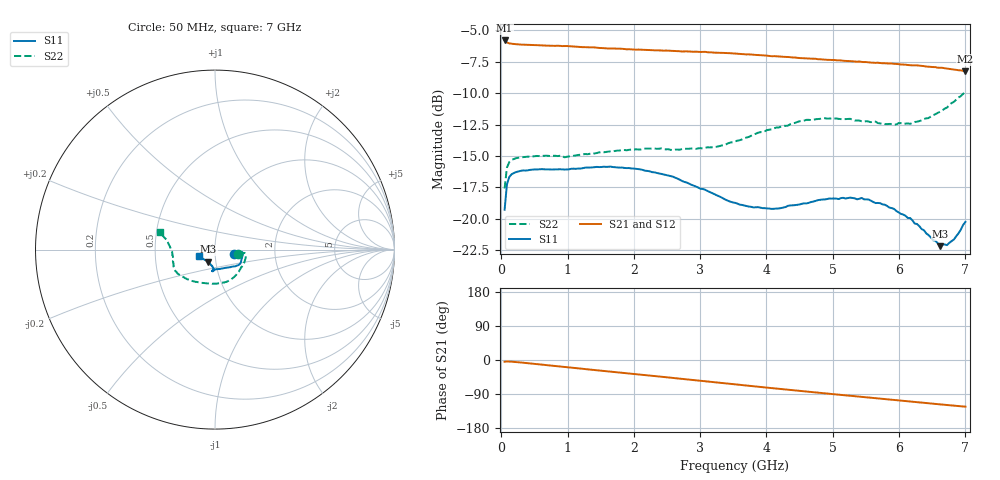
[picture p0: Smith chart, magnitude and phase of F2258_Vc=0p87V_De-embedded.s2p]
! Integrated Device Technology
! Corporate Headquarters
! 6024 Silver Creek Valley Road
! San Jose, CA 95138  USA
! Phone:  1-408-284-8200
! Toll Free:  1-800-223-1366
! Webpage:  http://www.idt.com/
! Timing and RF Division
! 515 Groton Road, Suite 102
! Westford, MA 01886-6024
! Device:  F2258
! Description: Voltage Variable RF Attenuator
! Frequency:  50.0 -  6000.00 MHz
! Package:  3x3 mm Thin QFN Plastic Package: 16 pin
! Ports:  2 RF, 2 DC
!  Pin  1  = NC
!  Pin  2  = NC
!  Pin  3  = RF2  = Port 2
!  Pin  4  = GND
!  Pin  5  = Vdd
!  Pin  6  = NC
!  Pin  7  = VCTRL
!  Pin  8  = NC
!  Pin  9  = GND
!  Pin 10  = RF1  = Port 1
!  Pin 11  = NC
!  Pin 12  = NC
!  Pin 13  = NC
!  Pin 14  = NC
!  Pin 15  = NC
!  Pin 16  = NC
! Vcntrl:  0.870 Volts
! Vdd:  +3.300 Volts
! Current:  1.145 mA
! Data:  The device was measured on a the F2258 evaluation board which has
!  individual transmission lines to the RF pins.  Data was collected
!  using a calibrated network analyzer.  The evaluation board was
!  de-embedded using a TRL calibration technique.
!  The reference plane is the edge of the package pin.
! Misc:  SN 10
!  Action Tracker AT0285
! Date Measured:  2014-12-10
! Date:  2016-01-13  MJV
! Note:
!  Integrated Device Technology supplies this data as a sample of measured
!  data at the package pin for this product.  Your particular data for this
!  product may vary.
!  Data was taken at 25 degrees C.
!  Integrated Device Technology reserves the right to change this data at anytime.
!Freq_(GHz)  S11M_(dB)  S11P_(deg)  S21M_(dB)  S21P_(deg)  S12M_(dB)  S12P_(deg)  S22M_(dB)  S22P_(deg)
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# GHz S dB R 50
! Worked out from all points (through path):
!   201 points, 50 MHz to 7 GHz, reference 50 ohm
!   highest |S21| = -5.80 dB at 50 MHz (marker M1); lowest = -8.3 dB at 7 GHz (marker M2)
!   group delay of S21, straight-line fit = 48.6 ps
!   lowest |S11| = -22.2 dB at 6.618 GHz (marker M3), VSWR 1.17, Z = 45.9 - j6.27 ohm
!   |S11| at or under -10 dB: start of sweep to end of sweep
!   |S22| runs from -17.6 to -9.9 dB; largest |S21 - S12| = 0.0028
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0.05  -19.29 -13.1  -5.80 -4.6  -5.78 -4.6  -17.60 -10.3
0.08475  -17.27 -6.9  -5.96 -3.9  -5.96 -3.9  -15.93 -6.6
0.1195  -16.69 -5.4  -6.03 -4.0  -6.03 -4.0  -15.50 -6.6
0.189  -16.36 -5.4  -6.08 -4.9  -6.08 -4.9  -15.25 -8.1
0.6755  -16.07 -13.7  -6.21 -13.3  -6.22 -13.3  -14.98 -23.5
0.9535  -16.09 -19.8  -6.25 -18.4  -6.25 -18.4  -15.11 -33.4
1.2315  -15.97 -23.7  -6.33 -23.4  -6.32 -23.4  -14.88 -42.2
1.6485  -15.85 -28.8  -6.44 -30.8  -6.42 -30.8  -14.64 -54.0
2.37825  -16.39 -35.9  -6.59 -43.5  -6.61 -43.5  -14.42 -73.8
2.58675  -16.65 -39.1  -6.62 -47.3  -6.65 -47.3  -14.53 -80.0
3.0385  -17.64 -47.6  -6.71 -55.4  -6.71 -55.4  -14.40 -96.1
3.525  -18.74 -63.1  -6.84 -64.2  -6.88 -64.2  -13.86 -115.4
4.081  -19.22 -83.8  -7.06 -74.2  -7.06 -74.2  -12.88 -134.6
4.7065  -18.64 -96.7  -7.25 -85.1  -7.30 -85.1  -12.12 -149.3
5.2625  -18.32 -97.3  -7.45 -94.4  -7.49 -94.3  -12.04 -158.3
5.43625  -18.35 -95.5  -7.51 -97.2  -7.53 -97.2  -12.24 -161.2
5.85325  -19.12 -93.8  -7.64 -104.2  -7.66 -104.2  -12.45 -169.7
6.166  -19.95 -96.1  -7.77 -109.4  -7.80 -109.4  -12.44 -176.9
6.61775  -22.19 -119.2  -7.97 -117.0  -7.98 -117.0  -11.48 171.0
6.722  -22.11 -129.1  -8.03 -118.8  -8.05 -118.8  -11.15 168.2
6.82625  -21.66 -139.6  -8.11 -120.5  -8.11 -120.5  -10.69 166.3
7  -20.26 -156.8  -8.25 -123.2  -8.25 -123.3  -9.88 162.7
